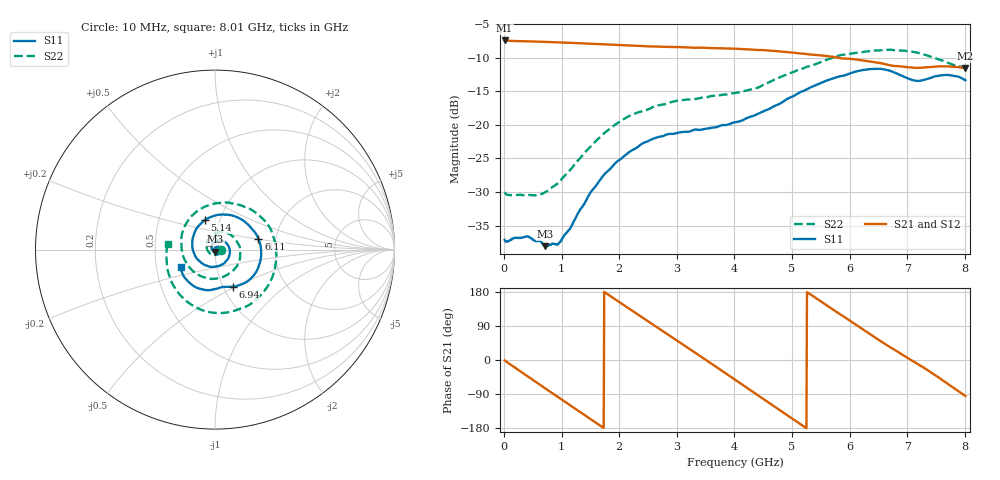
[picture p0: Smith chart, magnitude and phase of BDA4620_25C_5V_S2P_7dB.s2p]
!Agilent Technologies,E5071B,MY42404982,A.09.10
!Date: Wed May 06 08:59:35 2026
!Data & Calibration Information:
!Freq	S11:SOLT2(ON)	S21:SOLT2(ON)	S12:SOLT2(ON)	S22:SOLT2(ON)
# Hz S RI R 50
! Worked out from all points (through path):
!   801 points, 10 MHz to 8.01 GHz, reference 50 ohm
!   highest |S21| = -7.44 dB at 10 MHz (marker M1); lowest = -11.6 dB at 8.01 GHz (marker M2)
!   group delay of S21, straight-line fit = 283 ps
!   lowest |S11| = -38.1 dB at 710 MHz (marker M3), VSWR 1.03, Z = 50.2 - j1.24 ohm
!   |S11| at or under -10 dB: start of sweep to end of sweep
!   |S22| runs from -30.5 to -8.8 dB; largest |S21 - S12| = 0.0019
!   S11 on the Smith chart (normalised r, x): 10 MHz: 1.03, -0.00; 5.14 GHz: 0.85, +0.29; 6.11 GHz: 1.62, +0.21; 6.94 GHz: 1.11, -0.48; 8.01 GHz: 0.67, -0.14
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1e7  0.0139 -0.000801  0.4245 -0.00892  0.4251 -0.00924  0.0315 -0.00243
3.3e8  0.0129 -0.00682  0.3441 -0.2388  0.3445 -0.2395  0.0205 -0.0219
7.1e8  0.00215 -0.0123  0.112 -0.3989  0.112 -0.3995  -0.0113 -0.0295
9.6e8  -0.0099 -0.00889  -0.0726 -0.4042  -0.0729 -0.4049  -0.0345 -0.0151
1.35e9  -0.0202 0.0136  -0.3121 -0.2578  -0.312 -0.2579  -0.0469 0.0348
1.65e9  -0.0104 0.0365  -0.3943 -0.061  -0.3951 -0.0612  -0.0226 0.0765
1.94e9  0.0137 0.0504  -0.3687 0.1406  -0.369 0.1408  0.0271 0.0974
2.32e9  0.054 0.042  -0.1952 0.335  -0.1957 0.3354  0.1008 0.0716
2.68e9  0.0812 0.00534  0.0403 0.3799  0.0408 0.3802  0.1397 0.00228
3e9  0.077 -0.0399  0.2359 0.2971  0.2365 0.2969  0.1309 -0.076
3.39e9  0.0385 -0.0833  0.3671 0.0773  0.3675 0.0765  0.0526 -0.1486
3.69e9  -0.00952 -0.0958  0.3519 -0.1203  0.3517 -0.1212  -0.0404 -0.1599
4.01e9  -0.0669 -0.0803  0.2275 -0.2896  0.2269 -0.2903  -0.136 -0.1066
4.52e9  -0.1264 0.0134  -0.091 -0.3476  -0.0913 -0.3479  -0.1862 0.0745
5.14e9  -0.0553 0.1657  -0.3333 -0.067  -0.3337 -0.0666  0.0073 0.2581
5.35e9  0.00988 0.1923  -0.3279 0.0579  -0.3278 0.0583  0.1077 0.2553
5.74e9  0.1474 0.168  -0.2056 0.2446  -0.2055 0.2453  0.2759 0.1623
6.11e9  0.2418 0.0613  -0.016 0.3057  -0.0154 0.3062  0.3423 -0.0272
6.68e9  0.1872 -0.1723  0.2255 0.1636  0.2266 0.1633  0.2036 -0.2994
6.94e9  0.0977 -0.2069  0.2651 0.0549  0.2659 0.0544  0.065 -0.3507
7.51e9  -0.0492 -0.2249  0.2008 -0.183  0.2007 -0.1838  -0.2177 -0.2217
8.01e9  -0.1914 -0.0975  -0.0226 -0.2628  -0.023 -0.2638  -0.2645 0.0317
